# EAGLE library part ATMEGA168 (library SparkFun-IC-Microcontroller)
ATMEGA 168 Atmel 32-pin 8-bit micro, 16k flash. SparkFun Products SparkFun Serial Graphic LCD 128x64 (LCD-09351) SparkFun Graphic LCD Serial Backpack (LCD-09352) SparkFun Serial Graphic LCD 160x128 (LCD-08884)
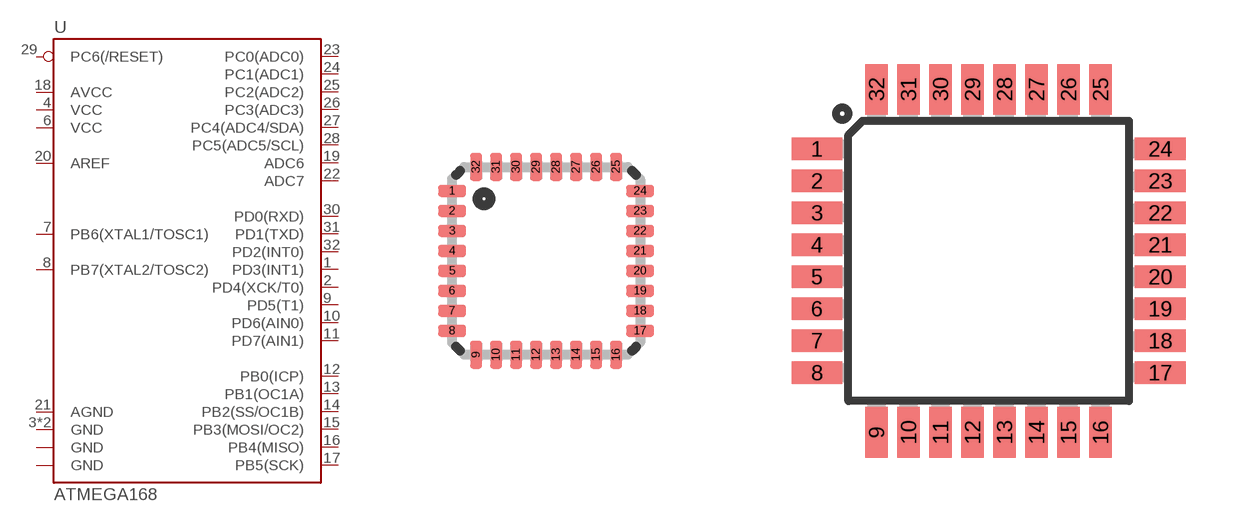
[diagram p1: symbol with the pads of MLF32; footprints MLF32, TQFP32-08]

Designator prefix U

## ATMEGA168MLF (PROD_ID: NA-XXXXX; VALUE: ATMEGA168)  [MLF32]
1  PD3(INT1)
2  PD4(XCK/T0)
3  GND
4  VCC
5  GND
6  VCC
7  PB6(XTAL1/TOSC1)
8  PB7(XTAL2/TOSC2)
9  PD5(T1)
10  PD6(AIN0)
11  PD7(AIN1)
12  PB0(ICP)
13  PB1(OC1A)
14  PB2(SS/OC1B)
15  PB3(MOSI/OC2)
16  PB4(MISO)
17  PB5(SCK)
18  AVCC
19  ADC6
20  AREF
21  AGND
22  ADC7
23  PC0(ADC0)
24  PC1(ADC1)
25  PC2(ADC2)
26  PC3(ADC3)
27  PC4(ADC4/SDA)
28  PC5(ADC5/SCL)
29  PC6(/RESET)
30  PD0(RXD)
31  PD1(TXD)
32  PD2(INT0)

## ATMEGA168 (PROD_ID: IC-08594; VALUE: ATMEGA168)  [TQFP32-08]
1  PD3(INT1)
2  PD4(XCK/T0)
3  GND
4  VCC
5  AGND
6  VCC
7  PB6(XTAL1/TOSC1)
8  PB7(XTAL2/TOSC2)
9  PD5(T1)
10  PD6(AIN0)
11  PD7(AIN1)
12  PB0(ICP)
13  PB1(OC1A)
14  PB2(SS/OC1B)
15  PB3(MOSI/OC2)
16  PB4(MISO)
17  PB5(SCK)
18  AVCC
19  ADC6
20  AREF
21  GND
22  ADC7
23  PC0(ADC0)
24  PC1(ADC1)
25  PC2(ADC2)
26  PC3(ADC3)
27  PC4(ADC4/SDA)
28  PC5(ADC5/SCL)
29  PC6(/RESET)
30  PD0(RXD)
31  PD1(TXD)
32  PD2(INT0)

## Footprint MLF32 (pad centres in mm)
32M1-A Micro Lead Frame package (MLF)
smd 0.7 x 0.3: 1 -2.35,1.75; 2 -2.35,1.25; 3 -2.35,0.75; 4 -2.35,0.25; 5 -2.35,-0.25; 6 -2.35,-0.75; 7 -2.35,-1.25; 8 -2.35,-1.75; 17 2.35,-1.75; 18 2.35,-1.25; 19 2.35,-0.75; 20 2.35,-0.25; 21 2.35,0.25; 22 2.35,0.75; 23 2.35,1.25; 24 2.35,1.75
smd 0.3 x 0.7: 9 -1.75,-2.35; 10 -1.25,-2.35; 11 -0.75,-2.35; 12 -0.25,-2.35; 13 0.25,-2.35; 14 0.75,-2.35; 15 1.25,-2.35; 16 1.75,-2.35; 25 1.75,2.35; 26 1.25,2.35; 27 0.75,2.35; 28 0.25,2.35; 29 -0.25,2.35; 30 -0.75,2.35; 31 -1.25,2.35; 32 -1.75,2.35

## Footprint TQFP32-08 (pad centres in mm)
Thin Plasic Quad Flat Package Grid 0.8 mm
smd 1.27 x 0.559: 1 -4.293,2.8; 2 -4.293,2; 3 -4.293,1.2; 4 -4.293,0.4; 5 -4.293,-0.4; 6 -4.293,-1.2; 7 -4.293,-2; 8 -4.293,-2.8; 17 4.293,-2.8; 18 4.293,-2; 19 4.293,-1.2; 20 4.293,-0.4; 21 4.293,0.4; 22 4.293,1.2; 23 4.293,2; 24 4.293,2.8
smd 0.559 x 1.27: 9 -2.8,-4.293; 10 -2,-4.293; 11 -1.2,-4.293; 12 -0.4,-4.293; 13 0.4,-4.293; 14 1.2,-4.293; 15 2,-4.293; 16 2.8,-4.293; 25 2.8,4.293; 26 2,4.293; 27 1.2,4.293; 28 0.4,4.293; 29 -0.4,4.293; 30 -1.2,4.293; 31 -2,4.293; 32 -2.8,4.293

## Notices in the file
Licensing: Creative Commons ShareAlike 4.0 International - https://creativecommons.org/licenses/by-sa/4.0
